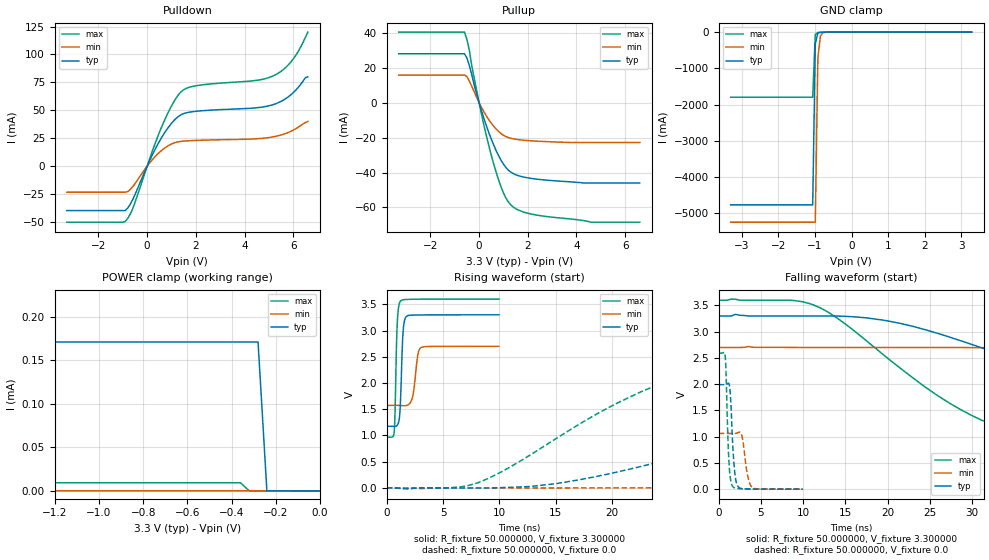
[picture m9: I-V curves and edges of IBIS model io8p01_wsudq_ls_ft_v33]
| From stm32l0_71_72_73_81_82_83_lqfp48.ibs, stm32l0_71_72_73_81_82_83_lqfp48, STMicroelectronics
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|   Model io8p01_wsudq_ls_ft_v33
[Model]  io8p01_wsudq_ls_ft_v33
Model_type I/O
Polarity   Non-Inverting
Enable   Active-Low
Vinl =   0.990000V
Vinh =   2.310000V
Vmeas =  1.650000V
Cref =   50.000000pF
Rref =   100.000000M
Vref =   0.0V
C_comp   2.653200pF   2.620200pF   2.695100pF
[Temperature Range]   25.000000   0.125000k   -40.000000
[Pullup Reference]   3.300000V   2.700000V   3.600000V
[Pulldown Reference]   0.0V   0.0V   0.0V
[POWER Clamp Reference]   3.300000V   2.700000V   3.600000V
[GND Clamp Reference]   0.0V   0.0V   0.0V
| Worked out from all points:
|   slope of the pulldown table from 0 to 0.495 V, typ, clamps not added: 22.6 ohm
|   slope of the pullup table from 0 to 0.495 V, typ, clamps not added: 23.9 ohm
|   GND clamp passes 1 mA (typ) near -0.64 V on its own axis
|   POWER clamp passes 1 mA (typ) near -2.99 V on its own axis
|   rising waveform, R_fixture 50.000000, V_fixture 3.300000: 20-80 % time 214ps typ, 362ps min, 177ps max; typ from 1.18 V to 3.3 V
|   rising waveform, R_fixture 50.000000, V_fixture 0.0: 20-80 % time 27.1ns typ, 59.7ns min, 13.6ns max; typ from 0 V to 1.99 V
|   falling waveform, R_fixture 50.000000, V_fixture 3.300000: 20-80 % time 24.2ns typ, 53.5ns min, 13.3ns max; typ from 3.3 V to 1.18 V
|   falling waveform, R_fixture 50.000000, V_fixture 0.0: 20-80 % time 398ps typ, 565ps min, 319ps max; typ from 1.99 V to 0 V
[Pulldown]
|Voltage   I(typ)   I(min)   I(max)
-3.3V     -39.83mA   -23.37mA   -50.2mA
-900mV    -39.83mA   -23.37mA   -49.53mA
-600mV    -30.28mA   -18.59mA   -38.45mA
500mV     22.11mA    12.28mA    30.1mA
1V        38.33mA    19.81mA    53.88mA
1.4V      46.1mA     22.18mA    66.72mA
2V        49.06mA    23.01mA    71.93mA
4.4V      52.05mA    24.38mA    76.53mA
5.2V      55.25mA    26.3mA     81.02mA
5.9V      63.83mA    31.17mA    93.18mA
6.2V      70.39mA    34.75mA    102.6mA
6.6V      80mA       40mA       120mA
[Pullup]
|Voltage   I(typ)   I(min)   I(max)
-3.3V     27.94mA    15.74mA    40.33mA
-600mV    27.94mA    15.74mA    40.33mA
-400mV    21.1mA     12.31mA    29.9mA
-300mV    15.86mA    9.288mA    20.96mA
200mV     -9.114mA   -5.293mA   -12.98mA
600mV     -24.28mA   -13.56mA   -35.12mA
1V        -35.19mA   -18.69mA   -51.62mA
1.2V      -38.61mA   -19.99mA   -56.78mA
1.4V      -40.59mA   -20.71mA   -59.71mA
2.2V      -43.48mA   -21.92mA   -63.91mA
4.6V      -46.01mA   -22.8mA    -68.41mA
6.6V      -46.01mA   -22.8mA    -68.41mA
[GND_clamp]
|Voltage   I(typ)   I(min)   I(max)
-3.3V     -4.766A    -5.244A    -1.797A
-1.06V    -4.766A    -5.244A    -1.797A
-990mV    -326.7mA   -5.244A    -68.05mA
-920mV    -29.09mA   -722.2mA   -11.16mA
-850mV    -6.797mA   -104.4mA   -6.682mA
-780mV    -3.554mA   -17.44mA   -4.265mA
-500mV    -58.08uA   -169.3uA   -34.1uA
3.28V     0A         0A         0A
[POWER_clamp]
|Voltage   I(typ)   I(min)   I(max)
-3.28V    3.05A      15.65uA    3.723A
-3.2V     3.05A      1.687uA    3.723A
-2.96V    269.4uA    209.1nA    3.723A
-2.92V    170.9uA    209.1nA    508.5mA
-2.8V     170.9uA    209.1nA    1.296mA
-2.76V    170.9uA    209.1nA    177.1uA
-2.72V    170.9uA    209.1nA    24.25uA
-2.68V    170.9uA    209.1nA    9.362uA
-360mV    170.9uA    209.1nA    9.362uA
-280mV    170.9uA    209.1nA    0A
-240mV    0A         209.1nA    0A
0V        0A         0A         0A
[Ramp]
| variable   typ   min   max
dV/dt_r  1.19496/27.05035n   0.63582/59.68353n   1.55568/13.54778n
dV/dt_f  1.27416/24.19555n   0.67080/53.42969n   1.57856/13.28247n
R_load = 50.000000
[Rising Waveform]
R_fixture= 50.000000
V_fixture= 3.300000
V_fixture_min= 2.700000
V_fixture_max= 3.600000
|time   V(typ)   V(min)   V(max)
0s        1.176V     1.573V     969.2mV
660.7ps   1.173V     1.574V     1.057V
940.9ps   1.197V     1.574V     3.149V
1.221ns   1.639V     1.571V     3.56V
1.441ns   2.929V     1.568V     3.586V
1.742ns   3.267V     1.571V     3.592V
2.302ns   3.294V     1.74V      3.596V
2.743ns   3.296V     2.51V      3.597V
3.083ns   3.297V     2.679V     3.598V
9.97ns    3.3V       2.7V       3.6V
[Rising Waveform]
R_fixture= 50.000000
V_fixture= 0.0
V_fixture_min= 0.0
V_fixture_max= 0.0
|time   V(typ)   V(min)   V(max)
0s        2.289nV    16.78nV    4.802nV
8.008ns   -307uV     -170.6uV   93.1mV
15.52ns   99.11mV    -129.4uV   1.005V
20.52ns   307.1mV    1.043mV    1.623V
26.53ns   623mV      8.208mV    2.147V
39.04ns   1.249V     79.32mV    2.523V
57.06ns   1.753V     281.4mV    2.584V
81.58ns   1.947V     593.9mV    2.592V
134.6ns   1.991V     957.8mV    2.593V
249.2ns   1.992V     1.062V     2.593V
[Falling Waveform]
R_fixture= 50.000000
V_fixture= 3.300000
V_fixture_min= 2.700000
V_fixture_max= 3.600000
|time   V(typ)   V(min)   V(max)
0s        3.3V       2.7V       3.6V
11.51ns   3.3V       2.7V       3.492V
19.52ns   3.22V      2.7V       2.56V
29.03ns   2.809V     2.698V     1.483V
39.54ns   2.219V     2.666V     1.054V
55.06ns   1.498V     2.528V     989.2mV
70.57ns   1.289V     2.322V     975.6mV
100.6ns   1.204V     1.903V     970mV
133.1ns   1.183V     1.699V     969.3mV
249.2ns   1.176V     1.573V     969.2mV
[Falling Waveform]
R_fixture= 50.000000
V_fixture= 0.0
V_fixture_min= 0.0
V_fixture_max= 0.0
|time   V(typ)   V(min)   V(max)
0s        1.992V     1.062V     2.593V
780.8ps   1.991V     1.062V     2.534V
1.221ns   2.007V     1.062V     528.8mV
1.421ns   1.733V     1.062V     176.6mV
1.642ns   941.5mV    1.062V     58.69mV
2.002ns   204.6mV    1.063V     17.73mV
2.462ns   26.75mV    1.087V     9.276mV
2.783ns   10.66mV    997.6mV    6.793mV
3.924ns   3.692mV    42.32mV    2.071mV
9.97ns    2.289nV    16.78nV    4.802nV
